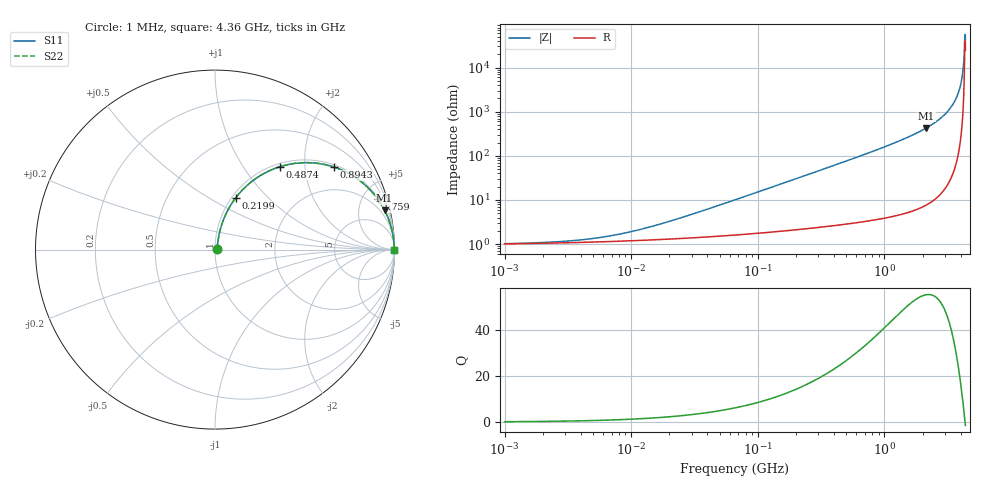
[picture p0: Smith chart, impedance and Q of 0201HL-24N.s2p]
# MHz  S  MA  R  50
!Freq  MagS11  AngS11  MagS21  AngS21  MagS12  AngS12  MagS22  AngS22
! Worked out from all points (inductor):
!   844 points, 1 MHz to 4.36 GHz, reference 50 ohm
!   read as one part in series: L = 24 nH near 27.21 MHz
!   highest Q = 55.5 at 2.147 GHz (marker M1), where L = 31.8 nH
!   self-resonance near 4.308 GHz
!   S11 on the Smith chart (normalised r, x): 1 MHz: 1.02, +0.00; 219.9 MHz: 1.04, +0.66; 487.4 MHz: 1.06, +1.49; 894.3 MHz: 1.07, +2.82; 1.759 GHz: 1.12, +6.35; 4.36 GHz: open
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1  0.01014 8.4  0.99 -0.1  0.99 -0.1  0.01014 8.4
4.06737  0.01244 28.8  0.9891 -0.3  0.9891 -0.3  0.01244 28.8
8.081435  0.01668 45.5  0.9884 -0.7  0.9884 -0.7  0.01668 45.5
16.3797  0.02741 61.4  0.9872 -1.4  0.9872 -1.4  0.02741 61.4
66.62232  0.09967 75.2  0.9794 -5.6  0.9794 -5.6  0.09967 75.2
219.8794  0.31 68.2  0.9307 -18.0  0.9307 -18.0  0.31 68.2
268.2947  0.3696 65.1  0.9085 -21.7  0.9085 -21.7  0.3696 65.1
487.4101  0.5868 51.9  0.7878 -35.9  0.7878 -35.9  0.5868 51.9
663.5247  0.7049 43.4  0.6877 -44.8  0.6877 -44.8  0.7049 43.4
894.331  0.8057 34.9  0.5718 -53.7  0.5718 -53.7  0.8057 34.9
1080.449  0.8581 29.6  0.4938 -59.1  0.4938 -59.1  0.8581 29.6
1759.348  0.9488 17.4  0.2986 -71.6  0.2986 -71.6  0.9488 17.4
2146.739  0.97 13.1  0.2261 -75.9  0.2261 -75.9  0.97 13.1
3010.966  0.9913 6.5  0.1129 -82.3  0.1129 -82.3  0.9913 6.5
3359.24  0.995 4.5  0.0784 -84.1  0.0784 -84.1  0.995 4.5
3673.951  0.997 2.9  0.05063 -85.2  0.05063 -85.2  0.997 2.9
3899.973  0.998 1.8  0.03228 -85.5  0.03228 -85.5  0.998 1.8
4058.328  0.9984 1.1  0.0201 -84.8  0.0201 -84.8  0.9984 1.1
4098.911  0.9985 1.0  0.01707 -84.3  0.01707 -84.3  0.9985 1.0
4223.112  0.9986 0.5  0.007994 -79.9  0.007994 -79.9  0.9986 0.5
4351.077  0.9987 -0.1  0.001783 44.1  0.001783 44.1  0.9987 -0.1
4360  0.9987 -0.1  0.002262 55.6  0.002262 55.6  0.9987 -0.1
